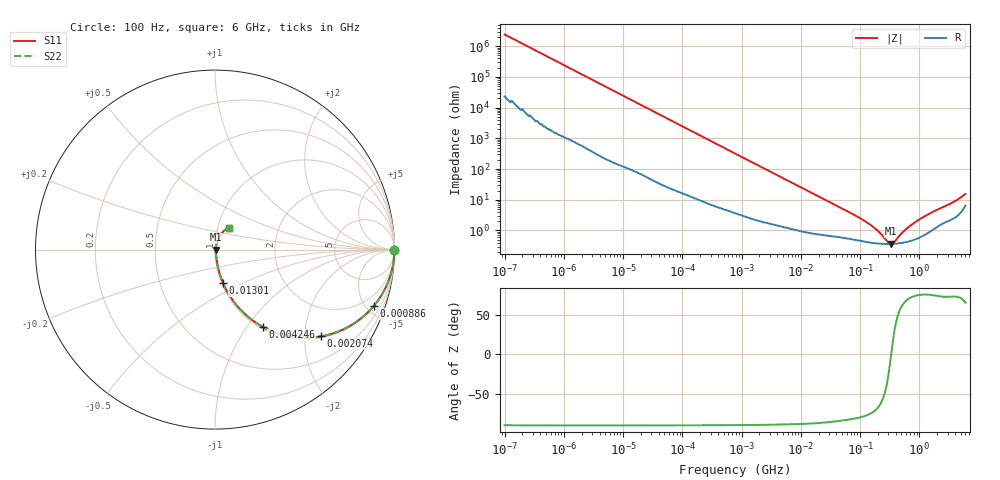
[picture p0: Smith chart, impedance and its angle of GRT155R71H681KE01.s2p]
!Murata Part Number: GRT155R71H681KE01
!These Parameters are Measured in Series Mode Connection
!Data Generated on Jun 19, 2026
!  o--ll--o
!Port1  Port2
!  o------o
!Operation Temp=25[degC], DC Bias Voltage=0[V]
!Freq. Start=100[Hz] Stop=6[GHz] 401[Steps]
# Hz S RI R 50
!Freq.(Hz) S11(Real) S11(Imag) S21(Real) S21(Imag) S12(Real) S12(Imag) S22(Real) S22(Imag)
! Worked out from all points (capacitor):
!   401 points, 100 Hz to 6 GHz, reference 50 ohm
!   read as one part in series: C = 659 pF near 109 Hz
!   lowest |Z| = 368 mohm at 326.7 MHz (marker M1)
!   series resonance near 334.7 MHz, so ESL is about 340 pH
!   S11 on the Smith chart (normalised r, x): 100 Hz: open; 886 kHz: 1.07, -5.62; 2.074 MHz: 1.04, -2.41; 4.246 MHz: 1.03, -1.19; 13.01 MHz: 1.02, -0.39; 6 GHz: 1.13, +0.28
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100  1 -4.15e-05  4e-07 4.15e-05  4e-07 4.15e-05  1 -4.15e-05
256  1 -0.000106  6e-07 0.000106  6e-07 0.000106  1 -0.000106
2008  1 -0.000825  4.6e-06 0.000825  4.6e-06 0.000825  1 -0.000825
40335  0.9996 -0.0164  0.000361 0.0164  0.000361 0.0164  0.9996 -0.0164
231233  0.9906 -0.0926  0.00939 0.0926  0.00939 0.0926  0.9906 -0.0926
774597  0.909 -0.282  0.091 0.282  0.091 0.282  0.909 -0.282
885955  0.8847 -0.3134  0.1153 0.3134  0.1153 0.3134  0.8847 -0.3134
1325623  0.7769 -0.4095  0.2231 0.4095  0.2231 0.4095  0.7769 -0.4095
2074311  0.5915 -0.4834  0.4085 0.4834  0.4085 0.4834  0.5915 -0.4834
4246196  0.2653 -0.4297  0.7347 0.4297  0.7347 0.4297  0.2653 -0.4297
6948629  0.1248 -0.3155  0.8752 0.3155  0.8752 0.3155  0.1248 -0.3155
1.300572e7  0.0445 -0.1858  0.9555 0.1858  0.9555 0.1858  0.0445 -0.1858
1.555665e7  0.0335 -0.1574  0.9665 0.1574  0.9665 0.1574  0.0335 -0.1574
3.64232e7  0.0112 -0.0694  0.9888 0.0694  0.9888 0.0694  0.0112 -0.0694
1.220122e8  0.00462 -0.0193  0.9954 0.0193  0.9954 0.0193  0.00462 -0.0193
1.909225e8  0.00387 -0.00974  0.9961 0.00974  0.9961 0.00974  0.00387 -0.00974
3.124326e8  0.00364 -0.00114  0.9964 0.00114  0.9964 0.00114  0.00364 -0.00114
3.267395e8  0.00365 -0.000398  0.9964 0.000398  0.9964 0.000398  0.00365 -0.000398
3.737127e8  0.00369 0.00184  0.9963 -0.00184  0.9963 -0.00184  0.00369 0.00184
5.847788e8  0.00422 0.00975  0.9958 -0.00975  0.9958 -0.00975  0.00422 0.00975
9.569533e8  0.00599 0.0206  0.994 -0.0206  0.994 -0.0206  0.00599 0.0206
6e9  0.0763 0.1219  0.9237 -0.1219  0.9237 -0.1219  0.0763 0.1219
